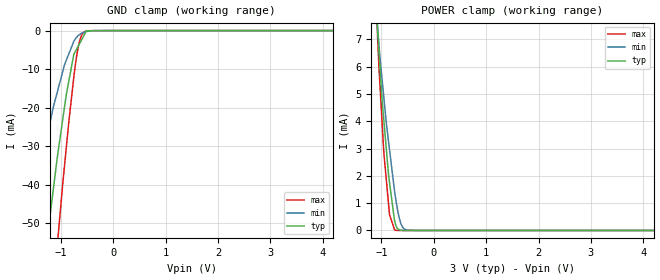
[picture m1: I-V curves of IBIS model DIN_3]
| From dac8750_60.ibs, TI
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|NOTES   Model TERM split into two Models TERM_3 and TERM_5
|   to accommodate the voltage range of 2.7V - 5.5V
|   TERM_3 operates in voltage range of 2.7 - 3 - 3.3
|   TERM_5 operates in voltage range of 4.5 - 5 - 5.5
|   DIN Models
[Model] DIN_3   |3V digital input
Model_type   Input
Vinl = 0.8
Vinh = 2
|   typ   min   max
|   (nom PVT)   (Fast PVT)   (slow PVT)
C_comp   2.090E-12   1.812E-12   2.388E-12
| Where   nom PVT is  Nominal Process, 3.0V, 36C
|   Fast PVT is Strong Process, 3.3V, -40C
|   Slow PVT is Weak Process, 2,7V, 134C
|C_comp - from L-C Tank method, L = 1nH, peak frequency
[Voltage Range]   3   2.7   3.3
|Operating Temperature   27   125   -40
|Junction Temperature
[Temperature Range]   36   134   -40
[Power Clamp Reference]   3   2.7   3.3
[GND Clamp Reference]   0   0   0
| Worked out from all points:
|   GND clamp passes 1 mA (typ) near -0.55 V on its own axis
|   POWER clamp passes 1 mA (typ) near -0.79 V on its own axis
[GND Clamp]
|   Voltage   I(typ)   I(min)   I(max)
-3V       -286.8mA   -179.8mA   -372mA
-1.628V   -99.46mA   -53.39mA   -146.1mA
-1.266V   -54.77mA   -27.78mA   -86.44mA
-1.148V   -41.82mA   -20.21mA   -68.27mA
-1.062V   -32.5mA    -15.77mA   -55.13mA
-894.7mV  -16.7mA    -7.717mA   -30.44mA
-750.8mV  -6.174mA   -2.803mA   -12.07mA
-716.9mV  -5.317mA   -2.077mA   -8.474mA
-632.3mV  -3.182mA   -957.1uA   -2.341mA
-544.5mV  -966.1uA   -379.9uA   -282.9uA
-484.3mV  -49.49uA   -183.5uA   -59.42uA
5.991V    0A         0A         0A
[POWER Clamp]
|   Voltage   I(typ)   I(min)   I(max)
-3V       86.79mA    70.34mA    106.2mA
-1.097V   8.12mA     8.09mA     8.184mA
-1.049V   6.659mA    6.875mA    6.076mA
-991.6mV  4.902mA    5.631mA    4.127mA
-950.1mV  3.963mA    4.81mA     2.779mA
-861.5mV  2.005mA    3.229mA    935.3uA
-844.5mV  1.756mA    2.96mA     581.3uA
-746.5mV  350uA      1.416mA    15.47uA
-694.2mV  77.22uA    788.3uA    2.737uA
-634.5mV  14.76uA    290.6uA    699.9nA
-498mV    2.158uA    9.225uA    58.7nA
5.991V    0A         0A         0A
